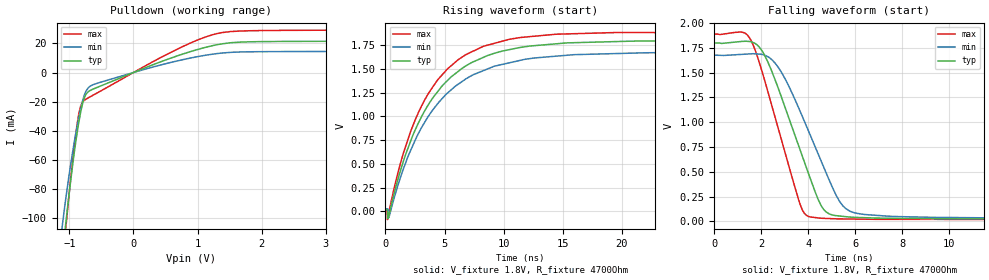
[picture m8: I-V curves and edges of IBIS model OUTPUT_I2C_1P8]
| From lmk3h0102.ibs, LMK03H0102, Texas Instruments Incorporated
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[Model]   OUTPUT_I2C_1P8
Model_type   Open_drain
Polarity   Non-Inverting
Vmeas = 0.9
Vref = 0
Cref = 10pF
Rref = 4700
|   typ   min   max
C_comp   0.7pF   0.5pF   0.9pF
[Voltage Range]   1.8   1.71   1.89
[Temperature Range]   45   125   -40
[Pullup Reference]   1.8   1.71   1.89
[Pulldown Reference]   0   0   0
[Power Clamp Reference]   1.8   1.71   1.89
[GND Clamp Reference]   0   0   0
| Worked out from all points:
|   slope of the pulldown table from 0 to 0.27 V, typ, clamps not added: 56.7 ohm
|   falling waveform, V_fixture 1.8V, R_fixture 4700Ohm: 20-80 % time 1.61ns typ, 1.8ns min, 1.35ns max; typ from 1.8 V to 0.021 V
|   rising waveform, V_fixture 1.8V, R_fixture 4700Ohm: 20-80 % time 4.7ns typ, 4.98ns min, 4.36ns max; typ from 0.021 V to 1.8 V
[Pulldown]
|   Voltage   I(typ)   I(min)   I(max)
-3.3V     -1.111A    -994.6mA   -1.235A
-1.181V   -155mA     -130.2mA   -166mA
-1.063V   -106.3mA   -88.93mA   -110.1mA
-1.013V   -87.04mA   -73.2mA    -87.67mA
-914.1mV  -52.02mA   -45.46mA   -46.91mA
-854.7mV  -34.77mA   -31.34mA   -28.74mA
-795.3mV  -21.66mA   -19.82mA   -20.37mA
-735.9mV  -14.64mA   -12.47mA   -18.18mA
16.5mV    299uA      212.7uA    413.8uA
1.214V    18.26mA    12.49mA    25.72mA
1.828V    21.11mA    14.25mA    28.71mA
6.6V      22.24mA    14.99mA    30.18mA
[Ramp]
R_load = 4700
|   typ   min   max
dV/dt_r   1.06746/4.66996e-09   0.989953/4.95337e-09   1.12446/4.34729e-09
dV/dt_f   1.06746/1.60821e-09   0.989884/1.79644e-09   1.12446/1.34602e-09
[Falling Waveform]
V_fixture = 1.8V
V_fixture_min = 1.71V
V_fixture_max = 1.89V
R_fixture = 4700Ohm
C_fixture = 0F
|   Time   V(typ)   V(min)   V(max)
0s        1.8V       1.678V     1.89V
1.128ns   1.815V     1.685V     1.912V
1.571ns   1.812V     1.691V     1.821V
2.058ns   1.71V      1.683V     1.49V
2.62ns    1.407V     1.587V     1.02V
3.832ns   598.8mV    1.01V      79.77mV
4.654ns   119.1mV    548.2mV    29.41mV
5.469ns   49.54mV    156.8mV    23.63mV
6.859ns   32.45mV    60.4mV     19.73mV
1.25us    20.9mV     27.8mV     15.9mV
[Rising Waveform]
V_fixture = 1.8V
V_fixture_min = 1.71V
V_fixture_max = 1.89V
R_fixture = 4700Ohm
C_fixture = 0F
|   Time   V(typ)   V(min)   V(max)
0s        20.9mV     27.8mV     15.9mV
122.6ps   19.52mV    27.26mV    13.29mV
169.3ps   9.388mV    27.06mV    -86.95mV
288.8ps   -43.25mV   -63.07mV   -12.96mV
1.506ns   524.8mV    444.3mV    609.6mV
2.857ns   949.5mV    838.1mV    1.061V
6.127ns   1.472V     1.338V     1.595V
11.3ns    1.725V     1.588V     1.83V
19.47ns   1.789V     1.663V     1.884V
1.25us    1.8V       1.678V     1.89V
